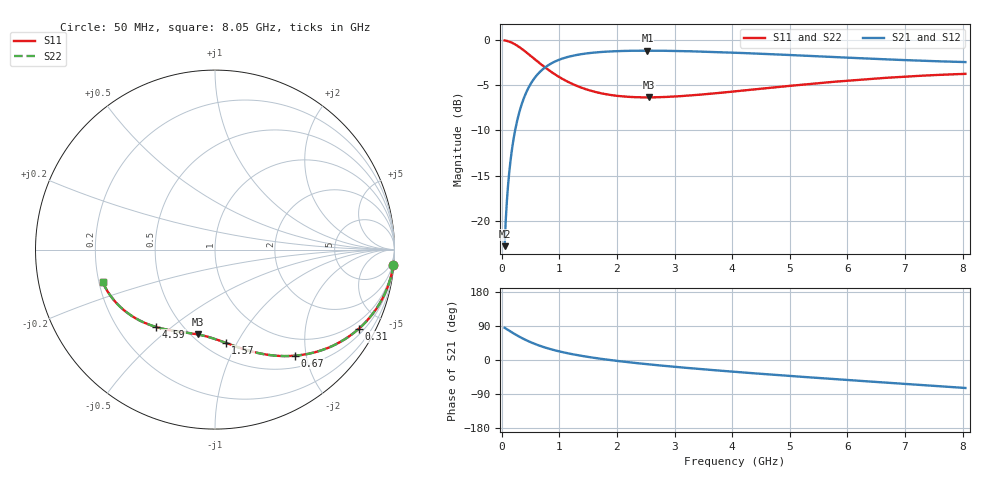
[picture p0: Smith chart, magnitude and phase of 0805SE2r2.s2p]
! AVX Thin Film Operation		Date: August 2001
! Description: Accu-P® Series, Thin Film, SMD, RF Capacitor
! Part Number: 08051J2R2ABT
! 50 MHz  -  8.05 GHz
! Serial Measurements
# mhz S db R 50
!	S11		S21		S12		S22
!	dB	Phase	dB	Phase	dB	Phase	dB	Phase
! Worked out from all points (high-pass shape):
!   401 points, 50 MHz to 8.05 GHz, reference 50 ohm
!   highest |S21| = -1.15 dB at 2.53 GHz (marker M1); lowest = -22.8 dB at 50 MHz (marker M2)
!   |S21| within 3 dB of the highest: 574 MHz to end of sweep
!   lowest |S11| = -6.3 dB at 2.55 GHz (marker M3), VSWR 2.86, Z = 27 - j33.2 ohm
!   |S11| at or under -10 dB: nowhere
!   |S22| runs from -6.3 to 0.0 dB; largest |S21 - S12| = 0
!   S11 on the Smith chart (normalised r, x): 50 MHz: 1, -23; 310 MHz: 0.70, -3.77; 670 MHz: 0.69, -1.80; 1.57 GHz: 0.63, -0.90; 4.59 GHz: 0.36, -0.44; 8.05 GHz: 0.22, -0.14
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50  -0.02 -4.9  -22.83 85.1  -22.83 85.1  -0.02 -4.9
70  -0.04 -6.9  -19.93 83.1  -19.93 83.1  -0.04 -6.9
130  -0.15 -12.7  -14.68 77.3  -14.68 77.3  -0.15 -12.7
170  -0.25 -16.5  -12.46 73.5  -12.46 73.5  -0.25 -16.5
230  -0.45 -22.0  -10.07 68.0  -10.07 68.0  -0.45 -22.0
310  -0.78 -28.8  -7.86 61.2  -7.86 61.2  -0.78 -28.8
470  -1.56 -40.9  -5.20 49.1  -5.20 49.1  -1.56 -40.9
670  -2.60 -52.9  -3.46 37.1  -3.46 37.1  -2.60 -52.9
830  -3.37 -60.5  -2.68 29.4  -2.68 29.4  -3.37 -60.6
990  -4.05 -66.9  -2.18 23.0  -2.18 23.0  -4.05 -67.0
1390  -5.27 -79.1  -1.53 10.8  -1.53 10.8  -5.27 -79.2
1570  -5.64 -83.5  -1.39 6.5  -1.39 6.5  -5.64 -83.5
1990  -6.15 -92.0  -1.21 -2.1  -1.21 -2.1  -6.15 -92.1
2530  -6.33 -101.1  -1.16 -11.1  -1.16 -11.1  -6.33 -101.1
2550  -6.33 -101.4  -1.16 -11.5  -1.16 -11.5  -6.33 -101.4
2730  -6.31 -104.0  -1.16 -14.1  -1.16 -14.1  -6.31 -104.1
3370  -6.07 -112.8  -1.24 -22.9  -1.24 -22.9  -6.07 -112.8
4050  -5.67 -121.1  -1.38 -31.2  -1.38 -31.2  -5.67 -121.2
4590  -5.32 -127.4  -1.52 -37.5  -1.52 -37.5  -5.32 -127.4
5390  -4.82 -136.1  -1.75 -46.3  -1.75 -46.3  -4.82 -136.2
6730  -4.14 -150.1  -2.13 -60.3  -2.13 -60.3  -4.14 -150.2
8050  -3.73 -163.7  -2.42 -73.8  -2.42 -73.8  -3.73 -163.7
